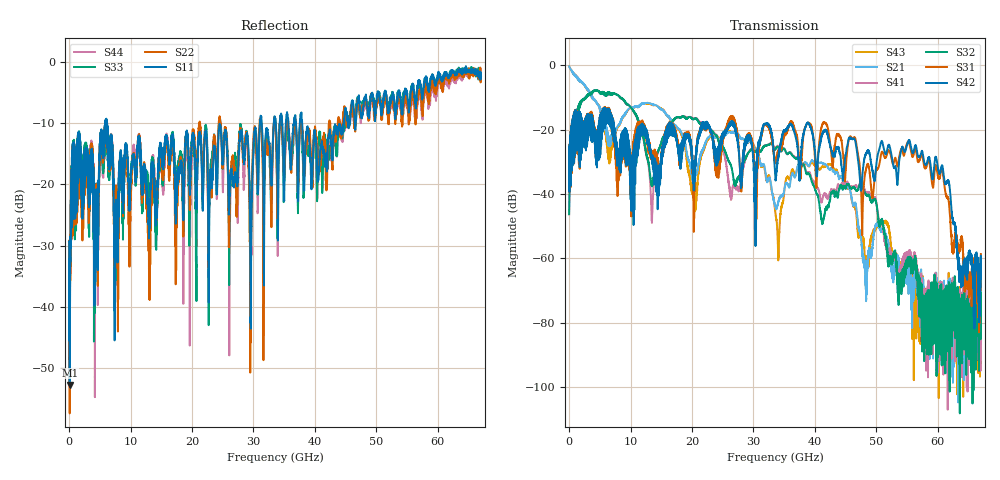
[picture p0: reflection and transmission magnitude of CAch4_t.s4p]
!Agilent Technologies,N5247A,US51170199,A.09.90.13
!Agilent N5247A: A.09.90.13
!Date: Wednesday, October 17, 2018 15:41:38
!Correction: S11(Full 4 Port(1,2,3,4))
!S12(Full 4 Port(1,2,3,4))
!S13(Full 4 Port(1,2,3,4))
!S14(Full 4 Port(1,2,3,4))
!S21(Full 4 Port(1,2,3,4))
!S22(Full 4 Port(1,2,3,4))
!S23(Full 4 Port(1,2,3,4))
!S24(Full 4 Port(1,2,3,4))
!S31(Full 4 Port(1,2,3,4))
!S32(Full 4 Port(1,2,3,4))
!S33(Full 4 Port(1,2,3,4))
!S34(Full 4 Port(1,2,3,4))
!S41(Full 4 Port(1,2,3,4))
!S42(Full 4 Port(1,2,3,4))
!S43(Full 4 Port(1,2,3,4))
!S44(Full 4 Port(1,2,3,4))
!S4P File: Measurements: <S11,S12,S13,S14>,
!<S21,S22,S23,S24>,
!<S31,S32,S33,S34>,
!<S41,S42,S43,S44>:
# Hz S  dB  R 50
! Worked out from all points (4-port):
!   6701 points, 10 MHz to 67 GHz, reference 50 ohm
!   strongest paths, dB at 10 MHz, 16.76 GHz, 33.51 GHz, 50.25 GHz, 67 GHz:
!     S42: -30.7, -20.6, -33.0, -27.6, -59.2
!     S31: -30.7, -20.3, -29.9, -32.1, -58.6
!     S32: -46.2, -17.6, -26.2, -46.7, -78.7
!     S41: -46.3, -17.6, -25.7, -46.1, -80.9
!     S21: -0.4, -18.0, -43.7, -49.5, -78.1
!     S43: -0.3, -18.1, -44.7, -49.4, -75.2
!   lowest |S11| = -52.8 dB at 99.99 MHz (marker M1), VSWR 1.00, Z = 49.8 - j0.109 ohm
!   |S11| at or under -10 dB: start of sweep to 5.858 GHz; 6.19 GHz to 31.05 GHz (24.86 GHz wide, 134 % of centre); 37.93 GHz to 44.65 GHz (6.722 GHz wide, 16.3 % of centre)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
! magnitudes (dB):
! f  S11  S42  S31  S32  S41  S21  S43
! 10 MHz  -29.3  -30.7  -30.7  -46.2  -46.3  -0.4  -0.3
! 99.99 MHz  -52.8  -26.8  -26.7  -36.9  -37.0  -0.8  -0.8
! 7.469 GHz  -28.7  -22.9  -25.0  -8.9  -8.9  -20.7  -21.3
! 13.48 GHz  -17.6  -28.0  -27.2  -37.5  -48.7  -12.1  -12.3
! 19.76 GHz  -18.7  -23.8  -23.8  -16.2  -16.1  -31.3  -36.4
! 55.3 GHz  -7.3  -23.3  -24.0  -61.3  -58.3  -63.1  -66.0
! 67 GHz  -2.6  -59.2  -58.6  -78.7  -80.9  -78.1  -75.2
